FUNCTION_BLOCK FB_Home_ByLimit
(*========================================
轴在任意位置回零功能块，无需考虑回零方向问题
默认回零方向：先负方向找原点,如果碰到负极限则改为正方向找原点

 By Swen & Richel	2017/2/8
==========================================*)
VAR_IN_OUT
	Axis				:	AXIS_REF;	(* B *)
END_VAR
VAR_INPUT
	Execute			:	BOOL;	(* B *)
	PosLimit		:BOOL;			(*正极限位信号*)
	NegLimit		:BOOL;			(*负极限位信号*)
	Position		:	LREAL			(* B *) := DEFAULT_HOME_POSITION;
	HomeingVelo		:LREAL	:=20;
	HomingMode		: 	MC_HomingMode;	(* V *)
	BufferMode		:	MC_BufferMode;		(* E *)
	Options			: 	ST_HomingOptions;	(* V *)	(* Beckhoff proprietary input *)
	bCalibrationCam 	: 	BOOL;	(* V *)	(* Beckhoff proprietary input *)


END_VAR
VAR_OUTPUT
	Done			:	BOOL;	(* B *)
	Busy			: 	BOOL;	(* E *)
	Active			: 	BOOL;	(* E *)
	CommandAborted	:	BOOL;	(* E *)
	Error			:	BOOL;	(* B *)
	ErrorID			:	UDINT;	(* E *)
END_VAR
VAR
	mcJog			:MC_Jog;
	mcHome			:MC_Home;
	HomeStep: INT;
END_VAR

IF  NOT Execute THEN
	mcJog.JogForward		:=FALSE;
	mcJog.JogBackwards		:=FALSE;
	mcHome.Execute			:=FALSE;
	done					:=FALSE;
	busy					:=FALSE;
	Error					:=FALSE;
	HomeStep				:=0;

END_IF


CASE HomeStep OF

0:
	busy	:=FALSE;
	Done	:=FALSE;
	IF 	Execute AND NOT Error  THEN

		IF	HomingMode  =MC_DefaultHoming  THEN  		 (*回零模式判断*)
			HomeStep	:=100;
		ELSE
			HomeStep	:=400;
		END_IF
		busy		:=TRUE;
		ErrorID		:=0;
	END_IF

100:
	mcJog.JogForward		:=FALSE;
	mcJog.JogBackwards		:=TRUE;		 (*先向负限位方向运动*)
	IF	NegLimit THEN
		mcJog.JogBackwards		:=FALSE;

		HomeStep	:=200;
	ELSIF  bCalibrationCam THEN
		mcJog.JogBackwards		:=FALSE;
		IF Axis.Status.NotMoving THEN
			HomeStep	:=400;
		END_IF
	ELSIF mcJog.Error THEN
			HomeStep	:=1000;

	END_IF

200:
	mcJog.JogBackwards		:=FALSE;
	mcJog.JogForward		:=TRUE;		(*向正限位方向运动*)

	IF	bCalibrationCam THEN
		HomeStep	:=300;
	ELSIF PosLimit THEN(*出错碰限位*)
		mcJog.JogForward		:=FALSE;
		HomeStep	:=1000;
	END_IF

300:

	mcJog.JogForward		:=FALSE;
	IF Axis.Status.NotMoving THEN
		HomeStep	:=400;
	END_IF


400:   (*调用回零功能块*)

	mcHome.Execute	:=TRUE;
	IF mcHome.Done AND AXIS.Status.Homed THEN
		done			:=TRUE;
		HomeStep	:=500;
	ELSIF AXIS.Status.Error THEN

		HomeStep	:=1000;
	END_IF

500:
	mcHome.Execute	:=FALSE;
	HomeStep		:=555;(*退出等待Execute下降沿*)

1000:
	Error			:=TRUE;
	IF	mcHome.ErrorID <> 0 THEN
		ErrorID			:=mcHome.ErrorID;
	ELSIF  mcJog.ErrorID <> 0 THEN
		ErrorID			:=mcJog.ErrorID;
	END_IF

	HomeStep		:=0;

END_CASE


Call_FB();

ACTION Call_FB:
mcJog
	(
	Velocity:=	HomeingVelo ,
	Mode:=		MC_JOGMODE_CONTINOUS ,
	Axis:=		Axis ,
	);

mcHome
	(
	Execute:= ,
	Position:=			Position ,
	HomingMode:= 		HomingMode,
	BufferMode:= 		BufferMode,
	Options:=			Options ,
	bCalibrationCam:=	bCalibrationCam ,
	Axis:=				Axis ,
	);
END_ACTION

END_FUNCTION_BLOCK
